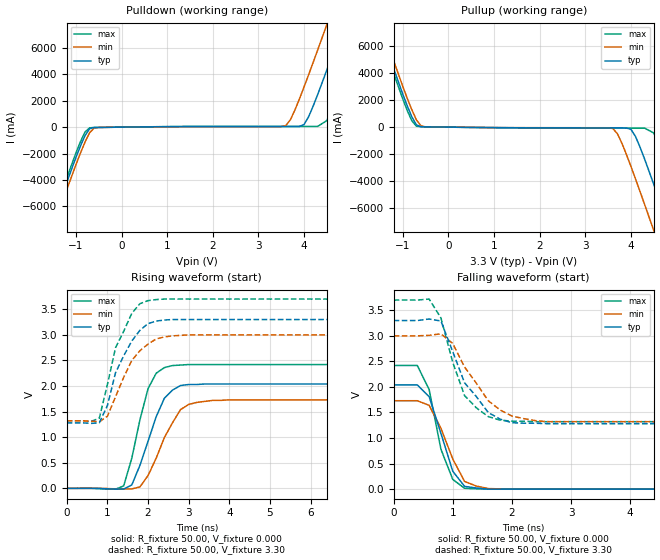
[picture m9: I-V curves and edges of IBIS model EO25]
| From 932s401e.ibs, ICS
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|   Model EO25
[Model]   EO25
Model_type   Output
Polarity   Non-Inverting
C_comp   2.50pF   2.00pF   3.00pF
[Temperature Range]   27.00   70.00   0.000
[Voltage Range]   3.30V   3.00V   3.70V
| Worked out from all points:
|   slope of the pulldown table from 0 to 0.495 V, typ, clamps not added: 24.5 ohm
|   slope of the pullup table from 0 to 0.495 V, typ, clamps not added: 25.6 ohm
|   rising waveform, R_fixture 50.00, V_fixture 0.000: 20-80 % time 551ps typ, 624ps min, 434ps max; typ from 0 V to 2.04 V
|   rising waveform, R_fixture 50.00, V_fixture 3.30: 20-80 % time 595ps typ, 643ps min, 559ps max; typ from 1.28 V to 3.3 V
|   falling waveform, R_fixture 50.00, V_fixture 0.000: 20-80 % time 335ps typ, 397ps min, 298ps max; typ from 2.04 V to 0 V
|   falling waveform, R_fixture 50.00, V_fixture 3.30: 20-80 % time 550ps typ, 601ps min, 399ps max; typ from 3.3 V to 1.28 V
[Pulldown]
| voltage   I(typ)   I(min)   I(max)
-3.3V     -24.68A    -25.34A    -24.36A
-1.7V     -8.95A     -9.49A     -8.61A
-1.5V     -7.01A     -7.56A     -6.67A
-900mV    -1.43A     -1.96A     -1.1A
-700mV    -120mA     -430mA     -51.82mA
3.6V      45.67mA    120mA      56.29mA
4V        200mA      3.05A      56.47mA
4.3V      2.48A      5.86A      57.28mA
4.5V      4.34A      7.78A      500mA
4.9V      8.18A      11.66A     3.99A
5.3V      12.09A     15.58A     7.84A
6.6V      24.93A     28.43A     20.64A
[Pullup]
| voltage   I(typ)   I(min)   I(max)
-3.3V     24.83A     25.38A     24.5A
-1.7V     9.1A       9.66A      8.74A
-1.5V     7.16A      7.73A      6.8A
-900mV    1.56A      2.11A      1.21A
-700mV    170mA      530mA      65.64mA
3.6V      -57.32mA   -95.98mA   -72.11mA
4V        -160mA     -2.9A      -73.07mA
4.3V      -2.36A     -5.71A     -74.4mA
4.5V      -4.22A     -7.63A     -430mA
4.9V      -8.06A     -11.52A    -3.89A
5.3V      -11.97A    -15.44A    -7.74A
6.6V      -24.83A    -28.31A    -20.55A
[Ramp]
| variable   typ   min   max
dV/dt_r   1.23/0.54n   1.04/0.62n   1.45/0.42n
dV/dt_f   1.21/0.48n   1.01/0.53n   1.43/0.39n
R_load = 50.00
[Rising Waveform]
R_fixture = 50.00
V_fixture = 0.000
V_fixture_min = 0.000
V_fixture_max = 0.000
| time   V(typ)   V(min)   V(max)
0s        0V         0V         0V
1.4ns     -13.18mV   -13.13mV   46.87mV
1.6ns     66.58mV    -10.81mV   590mV
1.8ns     450mV      27.26mV    1.34V
2ns       920mV      250mV      1.95V
2.2ns     1.4V       590mV      2.25V
2.4ns     1.76V      990mV      2.36V
2.8ns     2.01V      1.54V      2.41V
3.6ns     2.04V      1.72V      2.42V
10ns      2.04V      1.73V      2.42V
[Rising Waveform]
R_fixture = 50.00
V_fixture = 3.30
V_fixture_min = 3.00
V_fixture_max = 3.70
| time   V(typ)   V(min)   V(max)
0s        1.28V      1.32V      1.32V
800ps     1.28V      1.3V       1.37V
1ns       1.62V      1.41V      2.03V
1.2ns     2.26V      1.79V      2.75V
1.6ns     2.88V      2.5V       3.42V
1.8ns     3.09V      2.69V      3.61V
2ns       3.22V      2.82V      3.67V
2.4ns     3.29V      2.96V      3.7V
3ns       3.3V       3V         3.7V
10ns      3.3V       3V         3.7V
[Falling Waveform]
R_fixture = 50.00
V_fixture = 0.000
V_fixture_min = 0.000
V_fixture_max = 0.000
| time   V(typ)   V(min)   V(max)
0s        2.04V      1.73V      2.42V
400ps     2.04V      1.73V      2.42V
600ps     1.81V      1.64V      1.95V
800ps     1.09V      1.19V      780mV
1ns       350mV      590mV      190mV
1.2ns     53.76mV    150mV      16.35mV
1.4ns     21.22mV    59mV       6.1mV
1.6ns     -980uV     11.45mV    490uV
2ns       -160uV     -410uV     -130uV
10ns      2.14uV     -10.77uV   5.17uV
[Falling Waveform]
R_fixture = 50.00
V_fixture = 3.30
V_fixture_min = 3.00
V_fixture_max = 3.70
| time   V(typ)   V(min)   V(max)
0s        3.3V       3V         3.7V
600ps     3.33V      3.01V      3.72V
800ps     3.29V      3.04V      3.35V
1ns       2.69V      2.85V      2.48V
1.2ns     2.08V      2.39V      1.83V
1.6ns     1.5V       1.73V      1.42V
1.8ns     1.37V      1.55V      1.35V
2ns       1.3V       1.43V      1.33V
2.6ns     1.28V      1.32V      1.32V
10ns      1.28V      1.32V      1.32V
